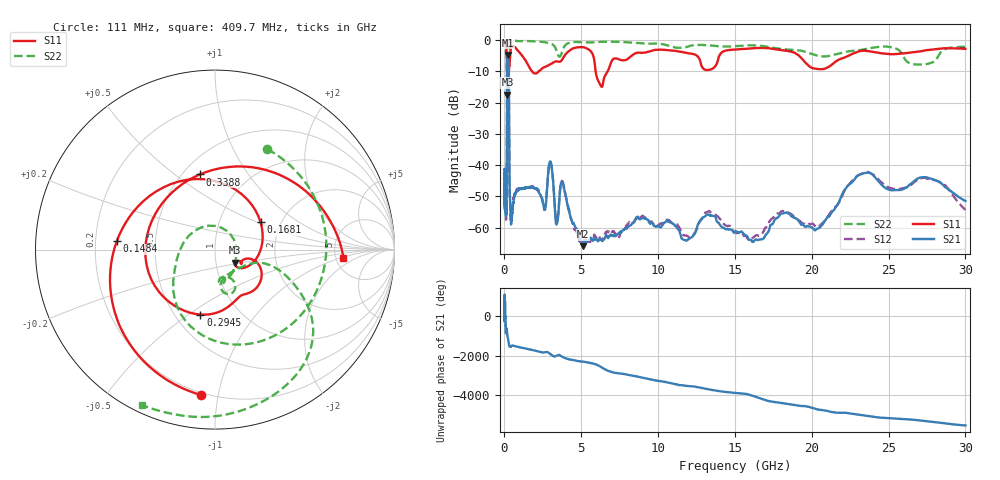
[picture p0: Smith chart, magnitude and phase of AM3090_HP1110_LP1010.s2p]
! Date/Time: Thu, Feb 28, 2019 2:09 PM
! Network Analyzer: Agilent Technologies E8364B Rev: A.07.50.67
! Sweep from 0.010 to 30.000 GHz, 1601 Points, Sweep Type: LOG
! Power Supply: 5.022 V, 0.002 A
# Hz S DB R 50
!freq MagS11 AngS11 MagS21 AngS21 MagS12 AngS12 MagS22 AngS22
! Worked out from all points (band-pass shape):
!   1601 points, 10 MHz to 30 GHz, reference 50 ohm
!   highest |S21| = -4.81 dB at 221.4 MHz (marker M1); lowest = -65.9 dB at 5.128 GHz (marker M2)
!   |S21| within 3 dB of the highest: 175.8 MHz to 276.1 MHz (100.4 MHz wide, 44.4 % of centre)
!   lowest |S11| = -17.4 dB at 192.5 MHz (marker M3), VSWR 1.31, Z = 62 - j9.09 ohm
!   |S11| at or under -10 dB: 166.3 MHz to 280.2 MHz (114 MHz wide, 51 % of centre); 1.793 GHz to 2.231 GHz (437.2 MHz wide, 21.7 % of centre); 5.93 GHz to 6.722 GHz (791.8 MHz wide, 12.5 % of centre)
!   |S22| runs from -18.5 to -0.2 dB; largest |S21 - S12| = 0.014
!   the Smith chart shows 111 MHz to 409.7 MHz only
!   S11 on the Smith chart (normalised r, x): 111 MHz: 0.19, -0.89; 148.4 MHz: 0.29, +0.04; 168.1 MHz: 1.57, +0.53; 294.5 MHz: 0.66, -0.56; 338.8 MHz: 0.60, +0.62; 409.7 MHz: 5.85, -1.14
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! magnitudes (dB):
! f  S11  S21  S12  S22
! 10 MHz  -0.2  -41.5  -42.4  -0.7
! 38.04 MHz  -0.3  -51.0  -50.8  -1.3
! 111 MHz  -1.8  -53.9  -54.5  -4.0
! 144.7 MHz  -4.5  -49.0  -49.0  -4.8
! 148.4 MHz  -5.2  -43.6  -44.0  -5.4
! 168.1 MHz  -10.6  -11.8  -11.8  -18.4
! 192.5 MHz  -17.4  -5.4  -5.4  -15.5
! 221.4 MHz  -15.8  -4.8  -4.8  -15.8
! 294.5 MHz  -8.6  -16.2  -16.1  -7.3
! 338.8 MHz  -7.4  -48.1  -47.8  -0.9
! 409.7 MHz  -2.9  -57.2  -56.4  -0.4
! 550.5 MHz  -2.0  -53.0  -51.9  -0.3
! 2.084 GHz  -10.7  -47.5  -47.4  -0.5
! 2.623 GHz  -8.7  -54.2  -53.8  -0.7
! 3.002 GHz  -7.7  -39.0  -39.0  -1.2
! 3.385 GHz  -6.8  -59.0  -57.8  -3.4
! 3.798 GHz  -6.0  -45.9  -45.4  -3.2
! 5.128 GHz  -2.3  -65.9  -64.6  -0.8
! 7.926 GHz  -6.3  -60.4  -59.4  -0.7
! 16.46 GHz  -2.6  -64.0  -62.4  -1.8
! 23.48 GHz  -3.5  -42.5  -42.4  -2.9
! 30 GHz  -2.8  -51.5  -54.3  -2.2
